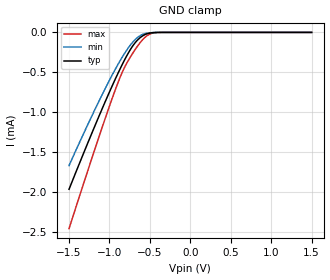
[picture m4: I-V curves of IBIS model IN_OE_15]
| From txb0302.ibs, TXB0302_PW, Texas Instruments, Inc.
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[Model]   IN_OE_15
Model_type  Input
Vinl=0.525
Vinh=0.975
| variable   typ   min   max
C_comp   0.35pF   0.25pF   0.44pF
[Temperature Range]   40   100   -40
| Ambient temperature   25   85   -40
[Voltage range]   1.5   1.35   1.65
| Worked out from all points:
|   GND clamp passes 1 mA (typ) near -1.11 V on its own axis
[GND Clamp]
| IN_OE_15
|   Voltage   I(typ)   I(min)   I(max)
-1.5V     -1.962mA   -1.665mA   -2.455mA
-1.285V   -1.425mA   -1.19mA    -1.782mA
-1.105V   -989.6uA   -808.7uA   -1.232mA
-970mV    -677.3uA   -540uA     -835.8uA
-875mV    -470uA     -365.9uA   -578.2uA
-800mV    -319uA     -242.3uA   -411.4uA
-700mV    -152.4uA   -108.6uA   -241.6uA
-625mV    -69.99uA   -43.64uA   -134.1uA
-550mV    -22.8uA    -13.11uA   -52.83uA
-480mV    -5.357uA   -3.255uA   -13.08uA
-385mV    -461.8nA   -298.9nA   -795.8nA
1.5V      93.72pA    297.1pA    7.149pA
